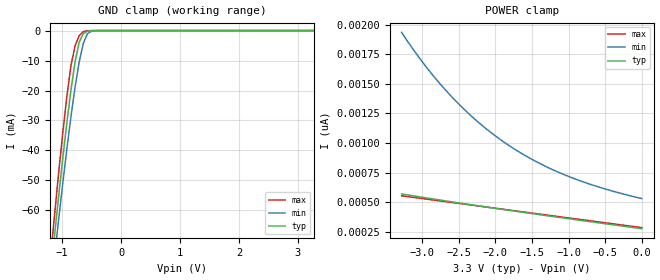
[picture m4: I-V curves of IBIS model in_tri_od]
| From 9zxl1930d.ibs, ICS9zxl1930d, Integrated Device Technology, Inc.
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|   Model in_tri_od
[Model]  in_tri_od
Model_type Input
Polarity   Non-Inverting
Vinl =   0.3000V
Vinh =   0.5000V
C_comp   1.4700pF   1.4700pF   1.4700pF
[Temperature Range]   25.0000   85.0000   -40.0000
[Voltage Range]   3.3000V   3.1350V   3.4650V
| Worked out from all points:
|   GND clamp passes 1 mA (typ) near -0.64 V on its own axis
[GND_clamp]
|Voltage   I(typ)   I(min)   I(max)
-3.3V     -537.9mA   -521.2mA   -558.4mA
-1.2V     -82.45mA   -88.85mA   -76.61mA
-1.13V    -68.84mA   -75.97mA   -62.02mA
-1.06V    -55.64mA   -63.44mA   -47.93mA
-920mV    -30.96mA   -39.73mA   -22.19mA
-850mV    -19.94mA   -28.84mA   -11.8mA
-780mV    -10.5mA    -18.94mA   -5.147mA
-710mV    -3.892mA   -10.51mA   -1.703mA
-640mV    -1.024mA   -4.276mA   -353.9uA
-570mV    -215.4uA   -1.063mA   -49.93uA
-430mV    -5.637uA   -33.74uA   -408.6nA
3.28V     273.7pA    551.6pA    269pA
[POWER_clamp]
|Voltage   I(typ)   I(min)   I(max)
-3.28V    568.6pA    1.935nA    553.1pA
-3.12V    552.7pA    1.789nA    540pA
-2.96V    537pA      1.655nA    526.8pA
-2.76V    517.8pA    1.503nA    510.4pA
-2.6V     502.5pA    1.393nA    497.3pA
-2.4V     483.8pA    1.269nA    480.9pA
-2.24V    469.1pA    1.179nA    467.8pA
-1.88V    436.5pA    1.006nA    438.3pA
-1.48V    401.2pA    854.8pA    405.5pA
-1.08V    366.6pA    737.3pA    372.7pA
-600mV    325.7pA    630pA      333.3pA
0V        275.4pA    529.8pA    284.1pA
